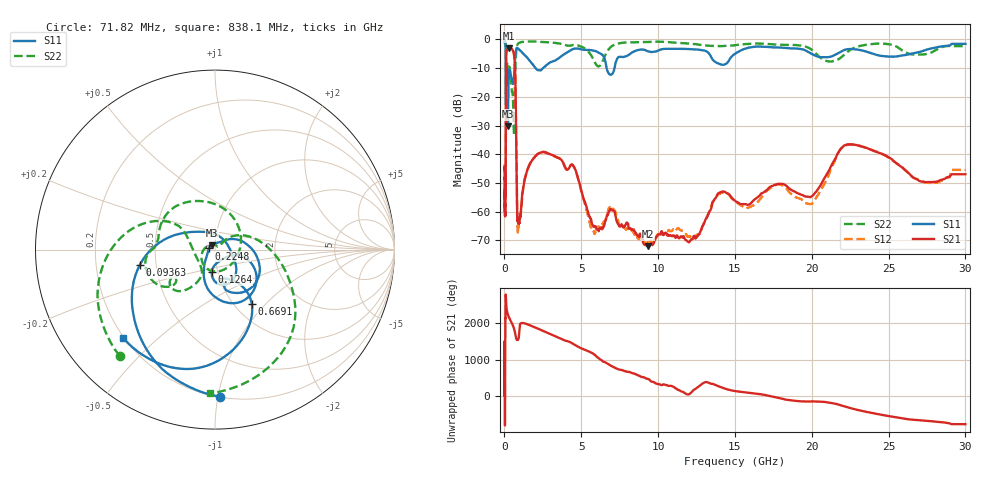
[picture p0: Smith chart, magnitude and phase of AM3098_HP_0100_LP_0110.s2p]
! Date/Time: Thu, Feb 28, 2019 8:35 AM
! Network Analyzer: Agilent Technologies E8364B Rev: A.07.50.67
! Sweep from 0.010 to 30.000 GHz, 1601 Points, Sweep Type: LOG
! Power Supply: 5.023 V, 0.002 A
# Hz S DB R 50
!freq MagS11 AngS11 MagS21 AngS21 MagS12 AngS12 MagS22 AngS22
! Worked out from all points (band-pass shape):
!   1601 points, 10 MHz to 30 GHz, reference 50 ohm
!   highest |S21| = -3.09 dB at 266.5 MHz (marker M1); lowest = -72.0 dB at 9.349 GHz (marker M2)
!   |S21| within 3 dB of the highest: 111 MHz to 640.6 MHz (529.6 MHz wide, 141 % of centre)
!   lowest |S11| = -30.2 dB at 229.3 MHz (marker M3), VSWR 1.06, Z = 48.1 + j2.32 ohm
!   |S11| at or under -10 dB: 176.8 MHz to 655.8 MHz (478.9 MHz wide, 115 % of centre); 2.031 GHz to 2.521 GHz (490.3 MHz wide, 21.5 % of centre); 6.648 GHz to 7.164 GHz (515.7 MHz wide, 7.47 % of centre)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
!   |S22| runs from -33.4 to -0.6 dB; largest |S21 - S12| = 0.012
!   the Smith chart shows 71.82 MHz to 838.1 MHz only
!   S11 on the Smith chart (normalised r, x): 71.82 MHz: 0.20, -1.02; 93.63 MHz: 0.40, -0.09; 126.4 MHz: 0.94, -0.24; 224.8 MHz: 0.94, +0.01; 669.1 MHz: 1.19, -0.84; 838.1 MHz: 0.20, -0.39
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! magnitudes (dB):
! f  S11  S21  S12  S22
! 10 MHz  -0.4  -45.3  -43.4  -0.6
! 38.04 MHz  -0.5  -59.7  -61.1  -0.9
! 71.82 MHz  -1.7  -51.0  -53.8  -2.0
! 93.63 MHz  -7.4  -21.7  -21.7  -8.6
! 126.4 MHz  -18.0  -4.6  -4.5  -10.3
! 144.7 MHz  -15.6  -3.8  -3.7  -10.7
! 184.9 MHz  -10.9  -3.6  -3.6  -8.0
! 224.8 MHz  -29.4  -3.2  -3.2  -9.4
! 229.3 MHz  -30.2  -3.2  -3.1  -9.5
! 266.5 MHz  -14.9  -3.1  -3.1  -9.8
! 550.5 MHz  -15.5  -3.9  -3.9  -20.4
! 620.7 MHz  -13.1  -5.3  -5.2  -33.4
! 669.1 MHz  -8.7  -8.0  -8.0  -20.7
! 838.1 MHz  -3.0  -61.9  -63.0  -1.9
! 2.084 GHz  -10.4  -40.3  -40.3  -0.8
! 4.436 GHz  -3.4  -43.7  -43.7  -2.0
! 5.754 GHz  -3.8  -64.9  -66.4  -6.6
! 7.926 GHz  -5.9  -63.9  -66.3  -1.1
! 9.349 GHz  -4.2  -72.0  -70.5  -0.9
! 19.8 GHz  -4.5  -54.8  -57.3  -3.0
! 22.67 GHz  -3.4  -36.6  -36.7  -3.2
! 30 GHz  -1.5  -47.0  -45.4  -2.4
